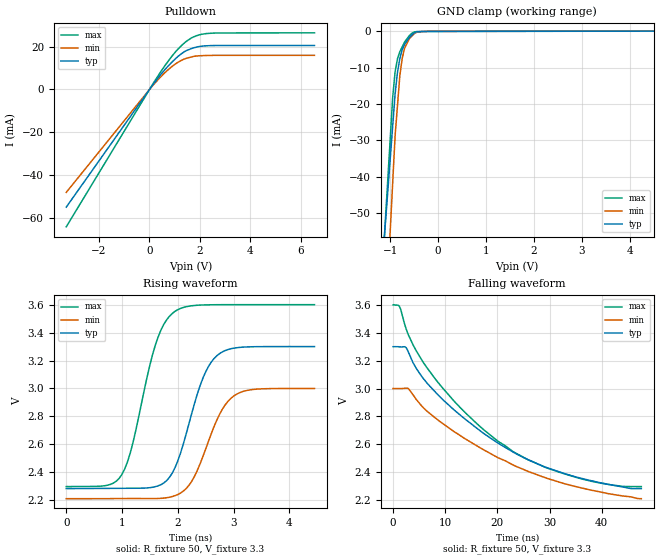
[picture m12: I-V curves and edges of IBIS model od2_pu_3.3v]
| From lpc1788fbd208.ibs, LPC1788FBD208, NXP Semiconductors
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[Model]   od2_pu_3.3v
Model_type I/O_open_drain
Vinl=9.900E-01
Vinh=2.310E+00
Vref=3.300E+00
Rref=2.000E+03
Cref=0.000E+00
Vmeas=1.650E+00
C_comp   5.160E-13   4.910E-13   5.420E-13
[Voltage Range]   3.300E+00   3.000E+00   3.600E+00
[POWER Clamp Reference]   3.300E+00   3.000E+00   3.600E+00
[GND Clamp Reference]   0.000E+00   0.000E+00   0.000E+00
[Pullup Reference]   3.300E+00   3.000E+00   3.600E+00
[Pulldown Reference]   0.000E+00   0.000E+00   0.000E+00
[Temperature Range]   25   85   -40
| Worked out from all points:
|   slope of the pulldown table from 0 to 0.495 V, typ, clamps not added: 64.9 ohm
|   GND clamp passes 1 mA (typ) near -0.54 V on its own axis
|   rising waveform, R_fixture 50, V_fixture 3.3: 20-80 % time 470ps typ, 490ps min, 462ps max; typ from 2.28 V to 3.3 V
|   falling waveform, R_fixture 50, V_fixture 3.3: 20-80 % time 20.8ns typ, 22.3ns min, 19.2ns max; typ from 3.3 V to 2.28 V
[GND Clamp]
-3.3V     -438.5mA   -646.2mA   -539.2mA
-950mV    -26.12mA   -41.76mA   -18.22mA
-900mV    -17.35mA   -28.9mA    -11.22mA
-850mV    -11.36mA   -20.52mA   -7.6mA
-800mV    -7.442mA   -12.15mA   -5.625mA
-750mV    -5.079mA   -7.409mA   -4.294mA
-700mV    -3.596mA   -4.64mA    -2.964mA
-600mV    -1.693mA   -2.032mA   -1.181mA
-500mV    -488.5uA   -682uA     -233.7uA
-400mV    -173.2uA   -129.9uA   -101.2uA
-200mV    -62.56uA   -47.1uA    -77.07uA
6.6V      35.04uA    32.39uA    35.06uA
[Pulldown]
-3.3V     -54.79mA   -47.91mA   -63.96mA
153mV     2.489mA    2.147mA    2.94mA
512.3mV   7.874mA    6.706mA    9.412mA
891.5mV   12.77mA    10.7mA     15.54mA
1.131V    15.41mA    12.66mA    18.82mA
1.43V     17.91mA    14.39mA    22.12mA
1.77V     19.45mA    15.47mA    24.58mA
2.269V    20.35mA    15.84mA    26.06mA
6.54V     20.51mA    15.9mA     26.38mA
[Rising Waveform]
R_fixture = 50
V_fixture = 3.3
V_fixture_min = 3
V_fixture_max = 3.6
0s        2.284V     2.211V     2.298V
1ns       2.285V     2.212V     2.386V
1.2ns     2.286V     2.212V     2.619V
1.6ns     2.297V     2.212V     3.314V
1.95ns    2.433V     2.233V     3.552V
2.3ns     2.893V     2.372V     3.594V
2.5ns     3.12V      2.567V     3.598V
2.7ns     3.234V     2.774V     3.6V
3.15ns    3.295V     2.976V     3.6V
4.45ns    3.3V       3V         3.6V
[Falling Waveform]
R_fixture = 50
V_fixture = 3.3
V_fixture_min = 3
V_fixture_max = 3.6
0s        3.3V       3V         3.6V
1.199ns   3.299V     3V         3.589V
2.447ns   3.295V     3.003V     3.433V
5.194ns   3.102V     2.888V     3.223V
8.241ns   2.969V     2.785V     3.061V
13.99ns   2.776V     2.636V     2.822V
20.13ns   2.609V     2.504V     2.622V
25.82ns   2.491V     2.407V     2.491V
32.62ns   2.394V     2.321V     2.392V
47.6ns    2.284V     2.211V     2.298V
[Ramp]
dV/dt_r   6.0988E-01/4.6880E-10   4.7340E-01/4.8990E-10   7.8133E-01/4.6000E-10
dV/dt_f   6.0988E-01/2.0795E-08   4.7340E-01/2.2268E-08   7.8133E-01/1.9147E-08
R_load = 50
